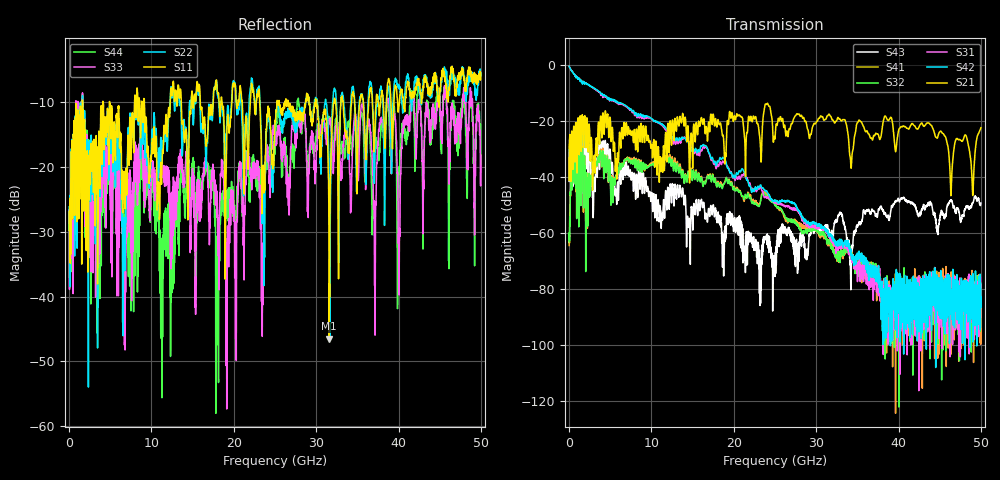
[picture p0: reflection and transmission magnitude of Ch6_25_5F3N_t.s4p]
!Agilent Technologies,N5247A,US51170199,A.09.90.13
!Agilent N5247A: A.09.90.13
!Date: Wednesday, December 16, 2015 09:41:17
!Correction: S11(Full 4 Port(1,2,3,4))
!S12(Full 4 Port(1,2,3,4))
!S13(Full 4 Port(1,2,3,4))
!S14(Full 4 Port(1,2,3,4))
!S21(Full 4 Port(1,2,3,4))
!S22(Full 4 Port(1,2,3,4))
!S23(Full 4 Port(1,2,3,4))
!S24(Full 4 Port(1,2,3,4))
!S31(Full 4 Port(1,2,3,4))
!S32(Full 4 Port(1,2,3,4))
!S33(Full 4 Port(1,2,3,4))
!S34(Full 4 Port(1,2,3,4))
!S41(Full 4 Port(1,2,3,4))
!S42(Full 4 Port(1,2,3,4))
!S43(Full 4 Port(1,2,3,4))
!S44(Full 4 Port(1,2,3,4))
!S4P File: Measurements: <S11,S12,S13,S14>,
!<S21,S22,S23,S24>,
!<S31,S32,S33,S34>,
!<S41,S42,S43,S44>:
# Hz S  dB  R 50
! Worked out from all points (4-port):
!   3201 points, 10 MHz to 50 GHz, reference 50 ohm
!   strongest paths, dB at 10 MHz, 12.51 GHz, 25 GHz, 37.5 GHz, 50 GHz:
!     S21: -41.3, -21.5, -26.3, -24.7, -22.4
!     S42: -0.4, -25.5, -48.4, -73.6, -83.2
!     S31: -0.4, -26.5, -49.4, -79.0, -79.3
!     S32: -63.2, -33.8, -50.2, -75.8, -80.5
!     S41: -64.5, -32.7, -49.7, -72.9, -81.7
!     S43: -41.6, -44.7, -75.6, -53.0, -49.4
!   lowest |S11| = -46.5 dB at 31.58 GHz (marker M1), VSWR 1.01, Z = 49.5 - j0.108 ohm
!   |S11| at or under -10 dB: 1.638 GHz to 4.102 GHz (2.464 GHz wide, 85.9 % of centre); 4.926 GHz to 7.953 GHz (3.027 GHz wide, 47 % of centre); 9.15 GHz to 12.29 GHz (3.135 GHz wide, 29.3 % of centre)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
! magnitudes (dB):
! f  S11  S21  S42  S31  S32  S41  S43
! 10 MHz  -29.8  -41.3  -0.4  -0.4  -63.2  -64.5  -41.6
! 650.5 MHz  -14.9  -25.4  -3.4  -3.4  -40.9  -40.0  -28.1
! 11.76 GHz  -12.2  -24.6  -22.5  -23.3  -33.9  -32.9  -45.5
! 23.18 GHz  -10.7  -26.5  -43.1  -43.5  -49.7  -49.3  -76.2
! 31.58 GHz  -46.5  -17.6  -61.1  -61.2  -63.3  -64.1  -60.2
! 46.38 GHz  -4.6  -46.5  -83.5  -91.0  -76.5  -82.6  -48.5
! 50 GHz  -5.6  -22.4  -83.2  -79.3  -80.5  -81.7  -49.4
